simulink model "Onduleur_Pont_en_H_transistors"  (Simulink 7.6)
settings: Solver=ode15s  StartTime=0.0  StopTime=N  RelTol=1e-3
InitFcn:
  | clc, close all
  | R=1e3; C=2500e-3/(5*pi);%1e-3/(5*pi)
  | 
  | R1=1e3
  | R2=R1;
  | 
  | N=0.002;
StopFcn:
  | load UI_Charge.mat
  | subplot 211
  | plotyy(x(1,:),x(2,:),x(1,:),x(3,:))
  | xlabel('temps')
  | title('Tension et courant - charge (R,L)')
  | axis([0 N -50 50])
  | 
  | grid
  | subplot 212
  | plot(x(1,:),x(4,:))
  | xlabel('temps')
  | title('Signal de gâchette PWM')
  | axis([0 N -0.2 1.2])
  | grid
  | 
  | 
  | delete *.mat
libraries: powerlib x10, fl_lib x3, nesl_utility x3, elec_lib x1

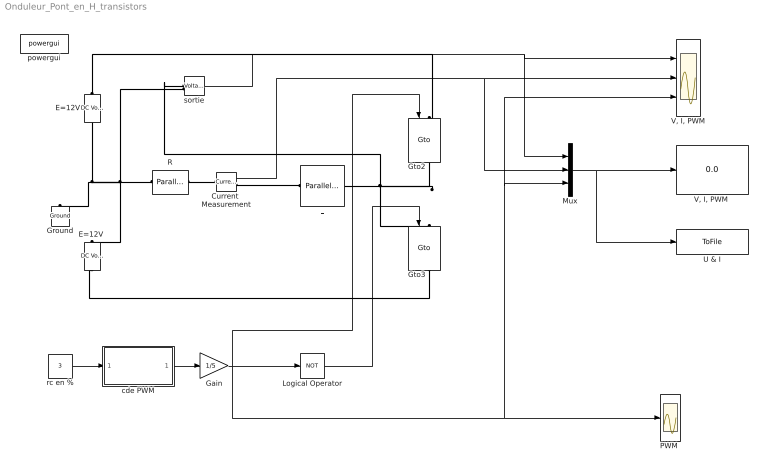
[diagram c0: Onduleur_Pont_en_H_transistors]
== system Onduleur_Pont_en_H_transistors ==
  Current  Measurement : powerlib/Measurements/Current Measurement  DialogController=POWERSYS.PowerSysDialog  SystemSampleTime=-1  PhasorSimulation=off  OutputType=Complex  PSBequivalent=0
  E=12V : powerlib/Electrical Sources/DC Voltage Source  DialogController=POWERSYS.PowerSysDialog  SystemSampleTime=-1  Amplitude=12  Measurements=None
  "E=12V " : powerlib/Electrical Sources/DC Voltage Source  DialogController=POWERSYS.PowerSysDialog  SystemSampleTime=-1  Amplitude=12  Measurements=None
  Gain : Gain  Gain=1/5
  Ground : powerlib/Elements/Ground  DialogController=POWERSYS.PowerSysDialog  PhysicalDomain=powersysdomain  SubClassName=unknown  LeftPortType=p1  RightPortType=p1  LConnTagsString=a
  Gto2 : powerlib/Power Electronics/Gto  DialogController=POWERSYS.PowerSysDialog  SystemSampleTime=-1  Ron=0.001  Lon=0  Vf=1  Tf=10e-6  Tt=20e-6  IC=0  Rs=1e5  Cs=inf  Measurements=on
  Gto3 : powerlib/Power Electronics/Gto  DialogController=POWERSYS.PowerSysDialog  SystemSampleTime=-1  Ron=0.001  Lon=0  Vf=1  Tf=10e-6  Tt=20e-6  IC=0  Rs=1e5  Cs=inf  Measurements=on
  L : powerlib/Elements/Parallel RLC Branch  DialogController=POWERSYS.PowerSysDialog  PhysicalDomain=powersysdomain  SubClassName=unknown  LeftPortType=p1  RightPortType=p1  LConnTagsString=a  RConnTagsString=__new0  BranchType=L  Resistance=1  Inductance=0.1  SetiL0=off  InitialCurrent=0  Capacitance=1e-6  Setx0=off  InitialVoltage=0  Measurements=None
  Logical Operator : Logic  Operator=NOT  AllPortsSameDT=off  OutDataTypeStr=boolean
  Mux : Mux  Inputs=3
  "PWM " : Scope
  R : powerlib/Elements/Parallel RLC Branch  DialogController=POWERSYS.PowerSysDialog  PhysicalDomain=powersysdomain  SubClassName=unknown  LeftPortType=p1  RightPortType=p1  LConnTagsString=a  RConnTagsString=__new0  BranchType=R  Resistance=10  Inductance=1.0  SetiL0=off  InitialCurrent=0  Capacitance=25e-06  Setx0=off  InitialVoltage=0  Measurements=Branch voltage and current
  U & I : ToFile  Filename=UI_Charge  MatrixName=x
  "V, I, PWM" : Scope  NumInputPorts=3
  "V, I, PWM " : Display
  cde PWM : Subsystem
  powergui : powerlib/powergui  SystemSampleTime=-1  SimulationMode=Continuous  SampleTime=0  frequency=60  SPID=off  DisableSnubberDevices=off  DisableRonSwitches=off  DisableVfSwitches=off  SwTol=0  Interpol=off  frequencyindice=0  echomessages=off  HookPort=off  DisplayEquations=off  FunctionMessages=off  EnableUseOfTLC=off  x0status=blocks  RestoreLinks=warning  ResistiveCurrentMeasurement=off  Frange=[0:2:500]  Ylog=off  Xlog=on  ShowGrid=off  save=off  variable=ZData  ZoomFFT=on  StartTime=0.0  cycles=1  DisplayStyle=1  fundamental=60  FreqAxis=off  MaxFrequency=1000  frequencyindicesteady=1  RmsSteady=1  display=off  Ts=0  methode=off
  rc en % : Constant  Value=3
  sortie : powerlib/Measurements/Voltage Measurement  DialogController=POWERSYS.PowerSysDialog  SystemSampleTime=-1  PhasorSimulation=off  OutputType=Complex  PSBequivalent=0
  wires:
  rc en %/1 -> cde PWM/1(" u")
  Mux/1 -> "V, I, PWM "/1, U & I/1
  cde PWM/1(" PWM") -> Gain/1
  sortie/1 -> "V, I, PWM"/1, Mux/1
  Current  Measurement/1 -> Mux/2, "V, I, PWM"/2
  Logical Operator/1 -> Gto3/1
  Gain/1 -> Logical Operator/1, Gto2/1, Mux/3, "V, I, PWM"/3, "PWM "/1
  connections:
  E=12V/LConn1 -- "E=12V "/RConn1 -- Ground/LConn1 -- R/RConn1 -- sortie/LConn2
  Gto3/RConn1 -- "E=12V "/LConn1
  R/LConn1 -- Current  Measurement/LConn1
  L/LConn1 -- Current  Measurement/RConn1
  Gto3/LConn1 -- Gto2/RConn1 -- L/RConn1 -- sortie/LConn1
  E=12V/RConn1 -- Gto2/LConn1

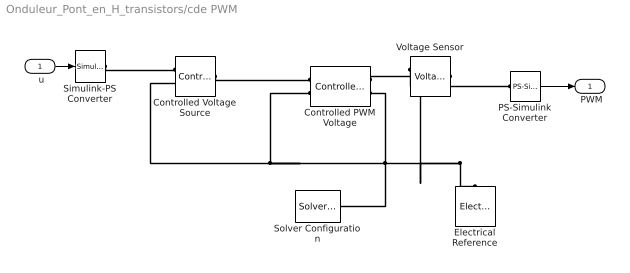
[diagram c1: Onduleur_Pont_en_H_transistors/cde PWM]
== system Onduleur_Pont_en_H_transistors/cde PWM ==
  " u" : Inport
  Controlled PWM Voltage : elec_lib/Actuators & Drivers/Drivers/Controlled PWM Voltage  DialogController=NetworkEngine.DynNeDlgSource  SystemSampleTime=-1  F=1000 Hz  Vmin=0 V  Vmax=5 V  Vm=5 V  pwm_or_av=1  current_Log=off  voltage_Log=off  power_Log=off  LocalVarNames=|current|voltage|power  LocalVarDescs=|Load current (A)|Load voltage (V)|Load power (W)  LocalVarLogging=[0 0 0]
  Controlled Voltage Source : fl_lib/Electrical/Electrical Sources/Controlled Voltage Source  DialogController=NetworkEngine.DynNeDlgSource  SystemSampleTime=-1  i_Log=off  v_Log=off  LocalVarNames=|i|v  LocalVarDescs=|i|v  LocalVarLogging=[0 0]
  Electrical Reference : fl_lib/Electrical/Electrical Elements/Electrical Reference  DialogController=NetworkEngine.DynNeDlgSource  SystemSampleTime=-1  i_Log=off  LocalVarNames=|i  LocalVarDescs=|i  LocalVarLogging=0
  PS-Simulink Converter : nesl_utility/PS-Simulink Converter  DialogController=NetworkEngine.DynNeUtilDlgSource  SystemSampleTime=-1  PhysicalDomain=network_engine_domain  LeftPortType=input  RightPortType=output  SubClassName=ps_output  Unit=1  AffineConversion=off
  Simulink-PS Converter : nesl_utility/Simulink-PS Converter  DialogController=NetworkEngine.DynNeUtilDlgSource  SystemSampleTime=-1  PhysicalDomain=network_engine_domain  LeftPortType=input  RightPortType=output  SubClassName=ps_input  Unit=1  AffineConversion=off  InputFilterTimeConstant=.001  UdotUserProvided=0
  Solver Configuration : nesl_utility/Solver Configuration  DialogController=NetworkEngine.DynNeUtilDlgSource  SystemSampleTime=-1  PhysicalDomain=network_engine_domain  LeftPortType=input  RightPortType=generic  SubClassName=solver  Accelerate=off  Profile=off  ResidualTolerance=1e-9  MaxNonlinIter=3  MaxModeIter=2  DoFixedCost=off  UseLocalSampling=off  DoDC=off  LinearAlgebra=Sparse  LocalSolverSampleTime=.001  LocalSolverChoice=NE_BACKWARD_EULER_ADVANCER  UseLocalSolver=off
  Voltage Sensor : fl_lib/Electrical/Electrical Sensors/Voltage Sensor  DialogController=NetworkEngine.DynNeDlgSource  SystemSampleTime=-1  i1_Log=off  v1_Log=off  LocalVarNames=|i1|v1  LocalVarDescs=|i1|v1  LocalVarLogging=[0 0]
  " PWM" : Outport
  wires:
  " u"/1 -> Simulink-PS Converter/1
  PS-Simulink Converter/1 -> " PWM"/1
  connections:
  Controlled Voltage Source/LConn1 -- Controlled PWM Voltage/LConn1
  Controlled PWM Voltage/RConn2 -- Electrical Reference/LConn1 -- Voltage Sensor/RConn2 -- Solver Configuration/RConn1 -- Controlled PWM Voltage/LConn2 -- Controlled Voltage Source/RConn2
  Controlled PWM Voltage/RConn1 -- Voltage Sensor/LConn1
  Simulink-PS Converter/RConn1 -- Controlled Voltage Source/RConn1
  Voltage Sensor/RConn1 -- PS-Simulink Converter/LConn1
